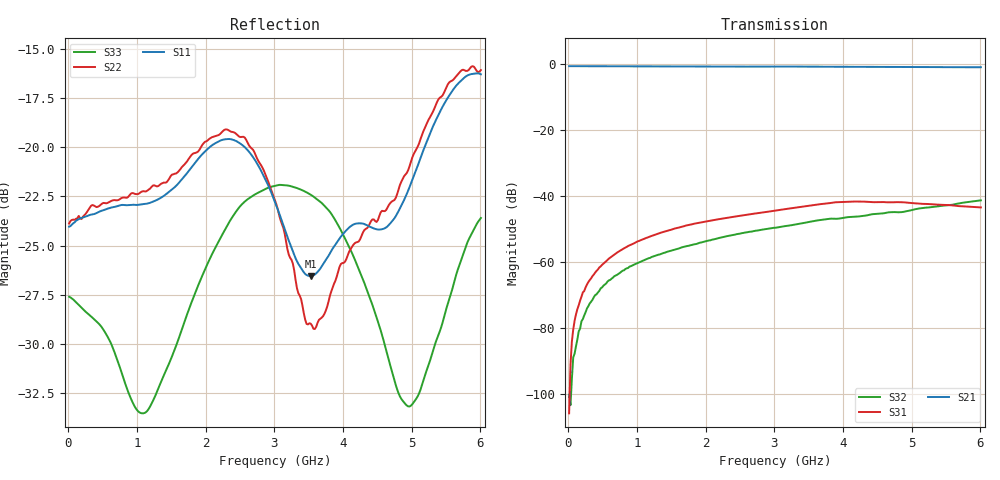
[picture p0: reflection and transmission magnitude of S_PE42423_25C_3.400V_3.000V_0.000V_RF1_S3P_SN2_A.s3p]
! Device ID: PE42423_Char_Units
! Serial: 2
! Insertion: A
! Temp: 25C
! VDD: 3.400
! Control_Hi: 3.000
! Control_Lo: 0.000
! Logic State: RF1
! ThroughPath: 2-1
! Port 1: RFC
! Port 2: RF1
! Port 3: RF2
! V1 = 3.00
! V2 = 0.00
! V3 = 0.00
! IDD: 1.364295e-04
! FILE NAME
! DATE 07-24-2013 19:14:31
! CORRECTED  DATA
#  Hz  S  RI  R  50
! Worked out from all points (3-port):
!   301 points, 10 MHz to 6.01 GHz, reference 50 ohm
!   strongest paths, dB at 10 MHz, 1.51 GHz, 3.01 GHz, 4.51 GHz, 6.01 GHz:
!     S21: -0.6, -0.7, -0.7, -0.8, -0.9
!     S31: -105.7, -50.0, -44.4, -41.8, -43.4
!     S32: -100.1, -56.4, -49.5, -45.3, -41.3
!   lowest |S11| = -26.5 dB at 3.53 GHz (marker M1), VSWR 1.10, Z = 53.7 - j3.23 ohm
!   |S11| at or under -10 dB: start of sweep to end of sweep
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1e7  0.0628 -3.97e-05  0.9287 -0.00284  5.22e-06 2.55e-07
     0.9301 -0.00297  0.064 -0.000303  -3.27e-08 -1.37e-06
     1.71e-06 -4.88e-06  -3.36e-06 -9.25e-06  -0.0417 0.000256
1.7e8  0.0658 -0.00403  0.9266 -0.0409  -4.09e-05 0.000256
       0.9278 -0.0402  0.066 -0.0021  -5.07e-05 9.86e-05
       -4.39e-05 0.000259  -4.66e-05 8.73e-05  -0.0394 0.00177
3.7e8  0.0669 -0.00954  0.9219 -0.0868  -9.5e-05 0.000657
       0.9231 -0.0863  0.0706 -0.00846  -9.67e-05 0.000274
       -9.3e-05 0.000645  -0.000106 0.000277  -0.0364 0.00331
8.1e8  0.07 -0.0137  0.904 -0.1851  -3.12e-05 0.00163
       0.9056 -0.1847  0.0732 -0.0141  -0.00016 0.000735
       -3.24e-05 0.00162  -0.00016 0.000738  -0.0249 0.00585
1.17e9  0.072 -0.00265  0.882 -0.2626  0.000192 0.00241
        0.8834 -0.2625  0.078 -0.00472  -0.000157 0.00114
        0.000196 0.00241  -0.000173 0.00114  -0.0139 0.0166
2.29e9  0.0908 0.0523  0.7764 -0.481  0.00152 0.00442
        0.7779 -0.4813  0.0976 0.053  -7.2e-05 0.00245
        0.00151 0.00441  -7.93e-05 0.00246  -0.00952 0.0614
3.01e9  0.0703 0.0177  0.6837 -0.6112  0.00262 0.00547
        0.6849 -0.6102  0.0694 0.0234  0.000183 0.00332
        0.00259 0.00547  0.000155 0.00333  -0.0412 0.0684
3.53e9  0.0363 -0.03  0.5963 -0.6943  0.00382 0.00618
        0.5985 -0.6933  0.0289 -0.0208  0.000297 0.00414
        0.00382 0.00619  0.000273 0.00411  -0.0588 0.0478
4.95e9  0.0653 -0.0419  0.3201 -0.8451  0.00674 0.00425
        0.323 -0.8448  0.067 -0.0562  0.000844 0.00598
        0.00674 0.00426  0.000823 0.00594  -0.000865 -0.0219
6.01e9  0.1517 -0.0226  0.0948 -0.8913  0.00606 0.00305
        0.0984 -0.891  0.1545 -0.0291  0.00185 0.00849
        0.00605 0.00304  0.00179 0.00847  0.0513 0.0417
